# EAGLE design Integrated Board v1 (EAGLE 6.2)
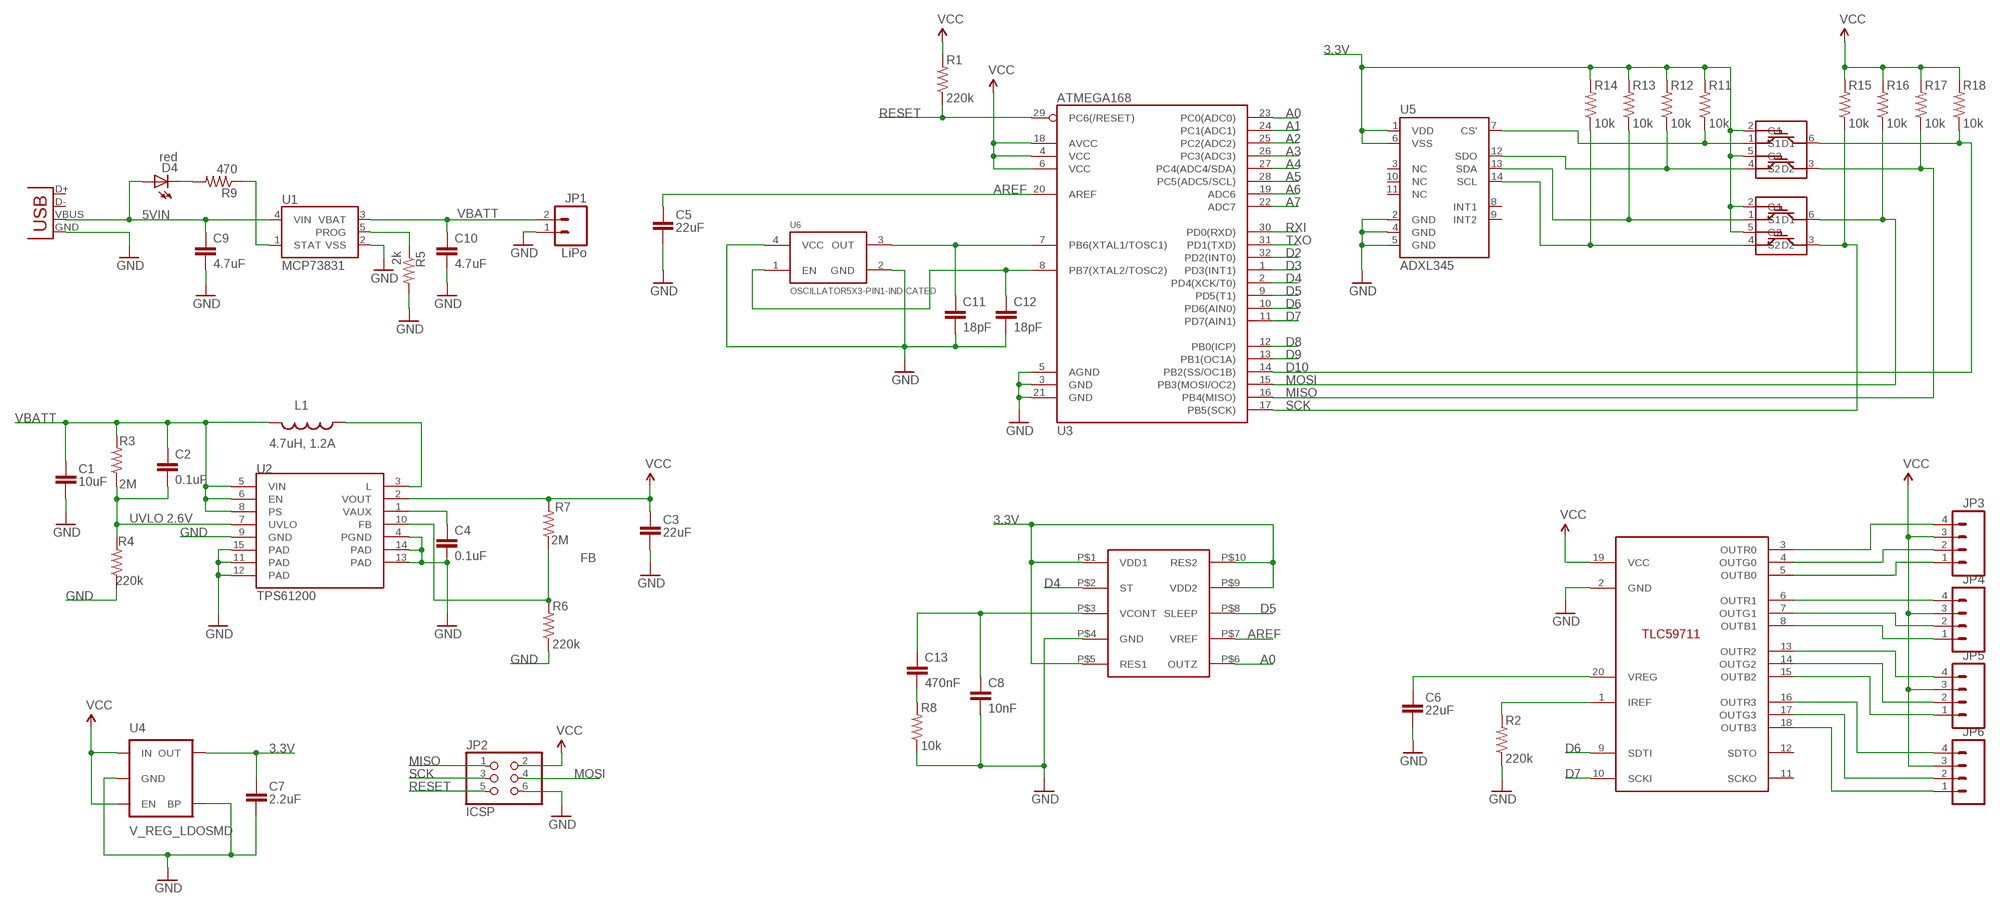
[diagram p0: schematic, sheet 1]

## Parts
C1  10uF  CAP0603  [0603]
C2  0.1uF  CAP0603-CAP  [0603-CAP]
C3  22uF  CAP0805  [0805]
C4  0.1uF  CAP0603-CAP  [0603-CAP]
C5  22uF  CAP0805  [0805]
C6  22uF  CAP0805  [0805]
C7  2.2uF  CAP0603  [0603]
C8  10nF  CAP0603-CAP  [0603-CAP]
C9  4.7uF  CAP0603-CAP  [0603-CAP]
C10  4.7uF  CAP0603-CAP  [0603-CAP]
C11  18pF  CAP0603-CAP  [0603-CAP]
C12  18pF  CAP0603-CAP  [0603-CAP]
C13  470nF  CAP0603-CAP  [0603-CAP]
D4  red  LED0603  [LED-0603]
JP1  LiPo  M02-JST-2MM-SMT  [JST-2-SMD]
JP2  ICSP  PINHD-2X3  [2X03]
JP3  M04PTH  [1X04]
JP4  M04PTH  [1X04]
JP5  M04PTH  [1X04]
JP6  M04PTH  [1X04]
L1  4.7uH, 1.2A  INDUCTOR.  [CDRH2D09]
R1  220k  RESISTOR0603-RES  [0603-RES]
R2  220k  RESISTOR0603-RES  [0603-RES]
R3  2M  RESISTOR0603-RES  [0603-RES]
R4  220k  RESISTOR0603-RES  [0603-RES]
R5  2k  RESISTOR0603-RES  [0603-RES]
R6  220k  RESISTOR0603-RES  [0603-RES]
R7  2M  RESISTOR0603-RES  [0603-RES]
R8  10k  RESISTOR0603-RES  [0603-RES]
R9  470  RESISTOR0603-RES  [0603-RES]
R11  10k  RESISTOR0603-RES  [0603-RES]
R12  10k  RESISTOR0603-RES  [0603-RES]
R13  10k  RESISTOR0603-RES  [0603-RES]
R14  10k  RESISTOR0603-RES  [0603-RES]
R15  10k  RESISTOR0603-RES  [0603-RES]
R16  10k  RESISTOR0603-RES  [0603-RES]
R17  10k  RESISTOR0603-RES  [0603-RES]
R18  10k  RESISTOR0603-RES  [0603-RES]
U1  MCP73831  [SOT23-5]
U2  TPS61200  [QFN-10_PAD]
U3  ATMEGA168  [TQFP32-08]
U4  V_REG_LDOSMD  [SOT23-5]
U5  ADXL345  [LGA14]
U6  OSCILLATOR5X3-PIN1-INDICATED  [CRYSTAL-OSC-SMD-5X3]
U$1  TLC59711  [TSSOP20]
U$2  2N7002DW  [SOT363]
U$3  2N7002DW  [SOT363]
U$4  LY3100ALH  [LGA10]
X1  USB-MICROB  [USB-MICROB]

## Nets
3.3V: C7.1 R11.2 R12.2 R13.2 R14.2 U4.5(OUT) U5.1(VDD) U5.6(VSS) U$2.2(G1) U$2.5(G2) U$3.2(G1) U$3.5(G2) U$4.P$1(VDD1) U$4.P$5(RES1) U$4.P$9(VDD2) U$4.P$10(RES2)
5VIN: C9.1 D4.A U1.4(VIN) X1.VBUS
A0: U3.23(PC0(ADC0)) U$4.P$6(OUTZ)
A1: U3.24(PC1(ADC1))
A2: U3.25(PC2(ADC2))
A3: U3.26(PC3(ADC3))
A4: U3.27(PC4(ADC4/SDA))
A5: U3.28(PC5(ADC5/SCL))
A6: U3.19(ADC6)
A7: U3.22(ADC7)
AREF: C5.1 U3.20(AREF) U$4.P$7(VREF)
D2: U3.32(PD2(INT0))
D3: U3.1(PD3(INT1))
D4: U3.2(PD4(XCK/T0)) U$4.P$2(ST)
D5: U3.9(PD5(T1)) U$4.P$8(SLEEP)
D6: U3.10(PD6(AIN0)) U$1.9(SDTI)
D7: U3.11(PD7(AIN1)) U$1.10(SCKI)
D8: U3.12(PB0(ICP))
D9: U3.13(PB1(OC1A))
D10: R18.1 U3.14(PB2(SS/OC1B)) U$2.6(D1)
FB: R6.2 R7.1 U2.10(FB)
GND: C1.2 C3.2 C4.2 C5.2 C6.2 C7.2 C8.2 C9.2 C10.2 C11.2 C12.2 JP1.1 JP2.6 R2.1 R4.1 R5.2 R6.1 R8.1 U1.2(VSS) U2.4(PGND) U2.9(GND) U2.11(PAD) U2.12(PAD) U2.13(PAD) U2.14(PAD) U2.15(PAD) U3.3(GND) U3.5(AGND) U3.21(GND) U4.2(GND) U4.4(BP) U5.2(GND) U5.4(GND) U5.5(GND) U6.2(GND) U6.4(VCC) U$1.2(GND) U$4.P$4(GND) X1.GND
MISO: JP2.1 R17.1 U3.16(PB4(MISO)) U$2.3(D2)
MOSI: JP2.4 R16.1 U3.15(PB3(MOSI/OC2)) U$3.6(D1)
N$1: C4.1 U2.1(VAUX)
N$2: L1.P$1 U2.3(L)
N$3: C11.1 U3.7(PB6(XTAL1/TOSC1)) U6.3(OUT)
N$5: C13.2 R8.2
N$6: C6.1 U$1.20(VREG)
N$7: R2.2 U$1.1(IREF)
N$8: D4.C R9.2
N$10: R11.1 U5.7(CS') U$2.1(S1)
N$11: R5.1 U1.5(PROG)
N$12: R12.1 U5.12(SDO) U$2.4(S2)
N$13: R13.1 U5.13(SDA) U$3.1(S1)
N$14: R9.1 U1.1(STAT)
N$15: R14.1 U5.14(SCL) U$3.4(S2)
N$16: JP4.4(B) U$1.6(OUTR1)
N$17: JP4.2(R) U$1.7(OUTG1)
N$18: JP4.1(COM) U$1.8(OUTB1)
N$19: JP5.4(B) U$1.13(OUTR2)
N$20: JP5.2(R) U$1.14(OUTG2)
N$21: JP5.1(COM) U$1.15(OUTB2)
N$22: JP6.4(B) U$1.16(OUTR3)
N$23: JP6.2(R) U$1.17(OUTG3)
N$24: JP6.1(COM) U$1.18(OUTB3)
N$25: JP3.1(COM) U$1.5(OUTB0)
N$26: JP3.2(R) U$1.4(OUTG0)
N$27: JP3.4(B) U$1.3(OUTR0)
N$28: C12.1 U3.8(PB7(XTAL2/TOSC2)) U6.1(EN)
N$30: C8.1 C13.1 U$4.P$3(VCONT)
RESET: JP2.5 R1.1 U3.29(PC6(/RESET))
RXI: U3.30(PD0(RXD))
SCK: JP2.3 R15.1 U3.17(PB5(SCK)) U$3.3(D2)
TXO: U3.31(PD1(TXD))
UVLO: C2.2 R3.1 R4.2 U2.7(UVLO)
VBATT: C1.1 C2.1 C10.1 JP1.2 L1.P$2 R3.2 U1.3(VBAT) U2.5(VIN) U2.6(EN) U2.8(PS)
VCC: C3.1 JP2.2 JP3.3(G) JP4.3(G) JP5.3(G) JP6.3(G) R1.2 R7.2 R15.2 R16.2 R17.2 R18.2 U2.2(VOUT) U3.4(VCC) U3.6(VCC) U3.18(AVCC) U4.1(IN) U4.3(EN) U$1.19(VCC)
Unconnected: U5.3(NC) U5.8(INT1) U5.9(INT2) U5.10(NC) U5.11(NC) U$1.11(SCKO) U$1.12(SDTO) X1.D+ X1.D-

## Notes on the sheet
- UVLO 2.6V

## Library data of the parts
C1 C3 C5-C7 = CH_passive:CAP: Capacitor
C2 C4 C8-C13 = SparkFun:CAP: Capacitor
D4 = SparkFun:LED: LEDs
JP1 = SparkFun:M02: Header 2
JP2 = SparkFun:PINHD-2X3: PIN HEADER
JP3-JP6 = SparkFun:M04: Header 4 Standard 4-pin 0.1" header. Use with straight break away headers (SKU : PRT-00116), right angle break away headers (PRT-00553), swiss pins (PRT-00743), machine pins (PRT-00117), and female headers (PRT-00115). Molex polarized connector foot print use with SKU : PRT-08231 with associated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
L1 = SparkFun:INDUCTOR: Inductors
R1-R9 R11-R18 = SparkFun:RESISTOR: Resistor
U1 = SparkFun:MCP73831: Microchip's MCP73831 Miniature single cell, fully integrated Li-Ion, Li-polymer charge management controller http://ww1.microchip.com/downloads/en/DeviceDoc/21984a.pdf
U2 = SparkFun:TPS61200: DC to DC Booster
U3 = SparkFun:ATMEGA168
U4 = SparkFun:V_REG_LDO: Voltage Regulator LDO Standard 150mA LDO voltage regulator in SOT-23 layout. Micrel part MIC5205. BP (by-pass) pin is used to lower output noise with 470pF cap.
U5 = SparkFun:ADXL345
U6 = SparkFun:OSCILLATOR
U$1 = SparkFun:TLC59711: TLC59711 RGB LED controller
U$2 U$3 = SparkFun:2N7002DW
U$4 = SparkFun:LY3100ALH
X1 = SparkFun:USB: USB Connectors USB-B-PTH is fully proven SKU : PRT-00139 USB-miniB is fully proven SKU : PRT-00587 USB-A-PCB is untested. USB-A-H is throughly reviewed, but untested. Spark Fun Electronics SKU : PRT-00437 USB-B-SMT is throughly reviewed, but untested. Needs silkscreen touching up. USB-A-S has not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

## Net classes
0 default: width 0.203 mm
1 vcc: width 0.254 mm

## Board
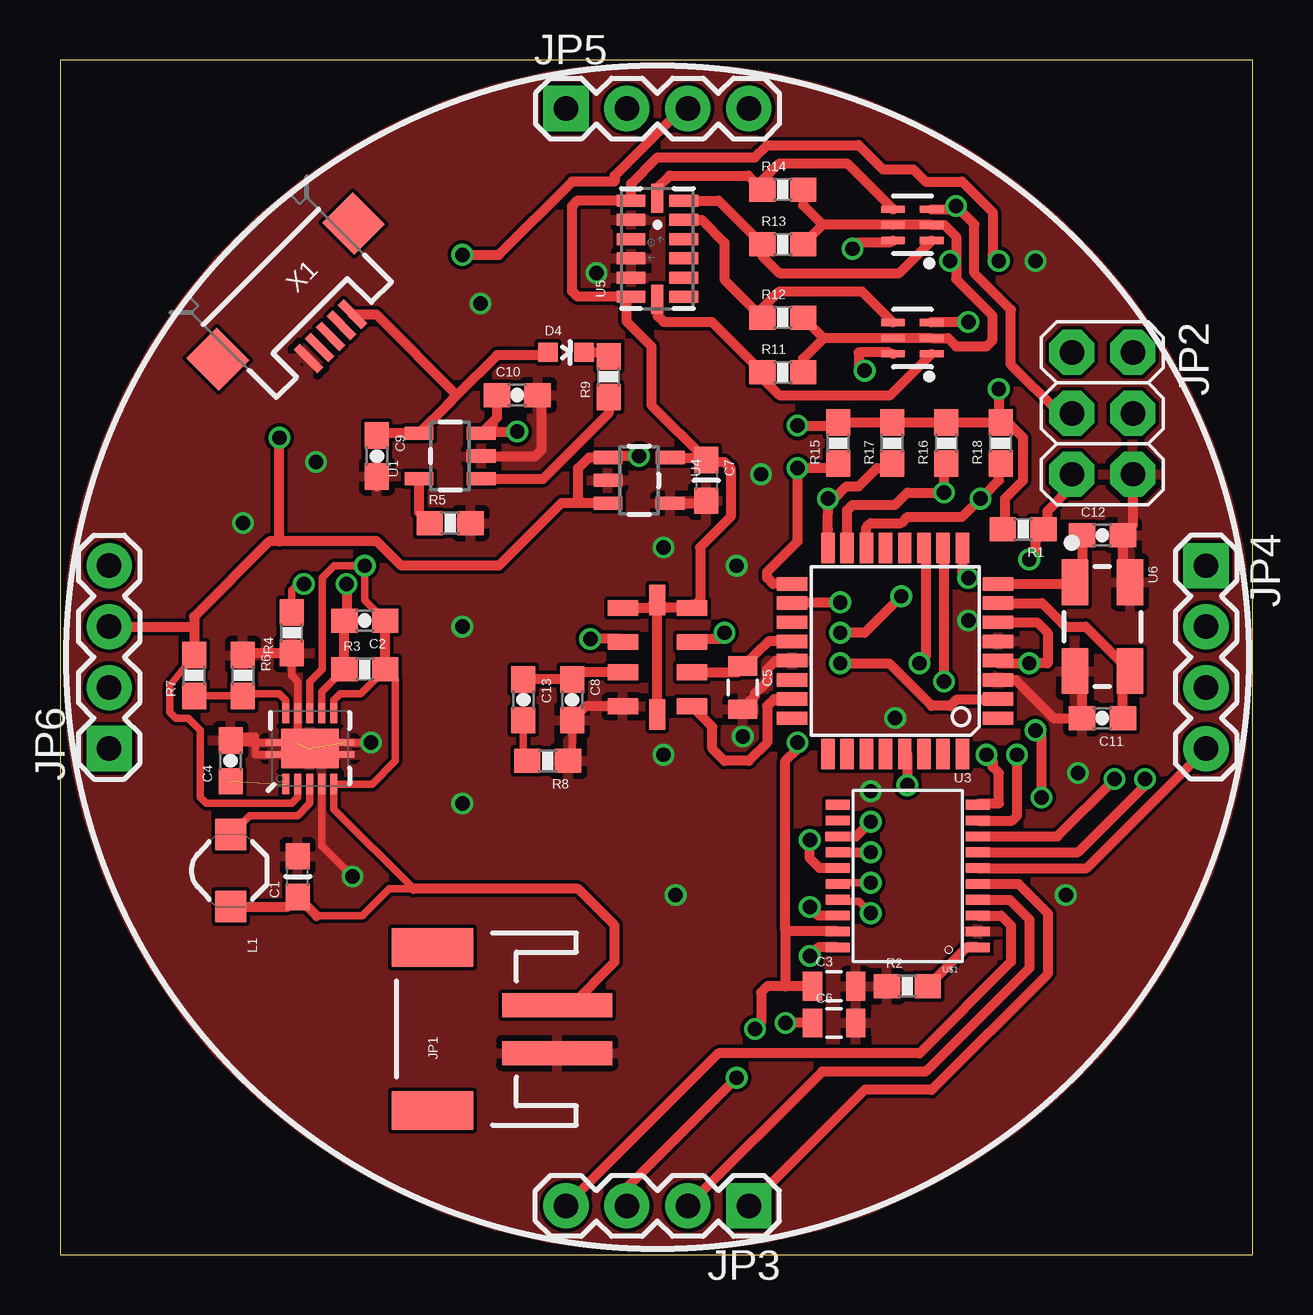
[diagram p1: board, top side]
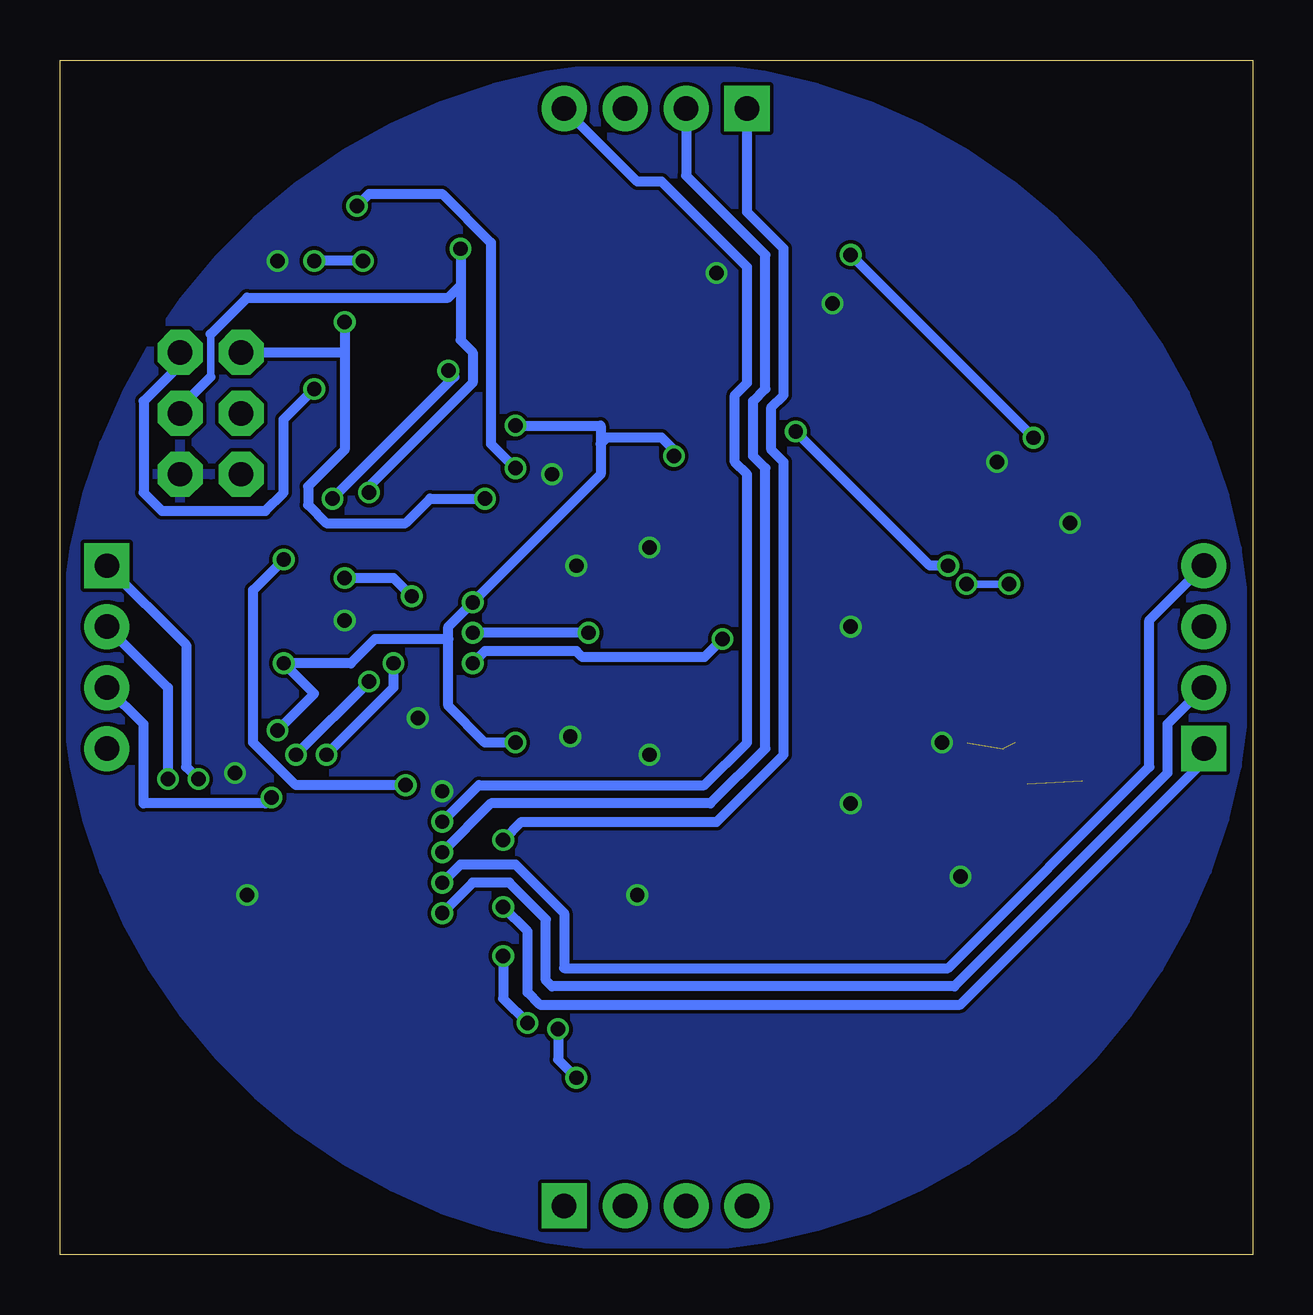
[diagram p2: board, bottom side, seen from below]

Size 49.71 x 49.77 mm. Coordinates in mm from the lower left corner, seen from the top.
Outline: 0,0 49.71,0 49.71,49.77 0,49.77 0,0
Copper layers (1*16): Top 0.035mm / dielectric 1.5mm / Bottom 0.035mm
Design rules: minimum track width 6mil, minimum drill 12mil, track to track 6mil, track to pad 6mil, pad to pad 6mil, via to via 6mil, smd to smd 0mil, copper to edge 10mil, drill to drill 10mil, minimum pad ring 10mil, minimum via ring 6mil, stop-mask expansion 2mil, vias tented up to drill 100mil, thermal gap 10mil

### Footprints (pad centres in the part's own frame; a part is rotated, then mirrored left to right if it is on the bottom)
0603 = smd 1.1 x 1: 1 -0.85,0; 2 0.85,0
0603-CAP = smd 1.1 x 1: 1 -0.85,0; 2 0.85,0
0805 = smd 0.8 x 1.2: 1 -0.9,0; 2 0.9,0
LED-0603 = smd 0.8 x 0.8: A 0,-0.75; C 0,0.75
JST-2-SMD = smd 1 x 4.6: 1 -1,-3.7; 2 1,-3.7 | smd 1.6 x 3.4: NC1 -3.4,1.5; NC2 3.4,1.5
2X03 = drill 1.016 pad 1.88 octagon: 1 -2.54,-1.27; 2 -2.54,1.27; 3 0,-1.27; 4 0,1.27; 5 2.54,-1.27; 6 2.54,1.27
1X04 = drill 1.016 pad 1.88 square: 1 0,0 | drill 1.016 pad 1.88: 2 2.54,0; 3 5.08,0; 4 7.62,0
CDRH2D09 = smd 1.3 x 1.3: P$1 -1.5,0; P$2 1.5,0
0603-RES = smd 1.1 x 1: 1 -0.85,0; 2 0.85,0
SOT23-5 = smd 0.55 x 1.2: 1 -0.95,-1.3; 2 0,-1.3; 3 0.95,-1.3; 4 0.95,1.3; 5 -0.95,1.3
QFN-10_PAD = smd 0.297 x 0.85: 1 -1,-1.475; 2 -0.5,-1.475; 3 0,-1.475; 4 0.5,-1.475; 5 1,-1.475; 6 1,1.475; 7 0.5,1.475; 8 0,1.475; 9 -0.5,1.475; 10 -1,1.475 | smd 0.7 x 0.28: 11 -1.5,0.25; 12 -1.5,-0.25; 13 1.5,0.25; 14 1.5,-0.25 | smd 2.4 x 1.65: 15 0,0
TQFP32-08 = smd 1.27 x 0.559: 1 -4.293,2.8; 2 -4.293,2; 3 -4.293,1.2; 4 -4.293,0.4; 5 -4.293,-0.4; 6 -4.293,-1.2; 7 -4.293,-2; 8 -4.293,-2.8; 17 4.293,-2.8; 18 4.293,-2; 19 4.293,-1.2; 20 4.293,-0.4; 21 4.293,0.4; 22 4.293,1.2; 23 4.293,2; 24 4.293,2.8 | smd 0.559 x 1.27: 9 -2.8,-4.293; 10 -2,-4.293; 11 -1.2,-4.293; 12 -0.4,-4.293; 13 0.4,-4.293; 14 1.2,-4.293; 15 2,-4.293; 16 2.8,-4.293; 25 2.8,4.293; 26 2,4.293; 27 1.2,4.293; 28 0.4,4.293; 29 -0.4,4.293; 30 -1.2,4.293; 31 -2,4.293; 32 -2.8,4.293
LGA14 = smd 0.5 x 1.2: 1 2,1.1; 2 1.2,1.1; 3 0.4,1.1; 4 -0.4,1.1; 5 -1.2,1.1; 6 -2,1.1; 8 -2,-1.1; 9 -1.2,-1.1; 10 -0.4,-1.1; 11 0.4,-1.1; 12 1.2,-1.1; 13 2,-1.1 | smd 1.2 x 0.5: 7 -2.1,0; 14 2.1,0
CRYSTAL-OSC-SMD-5X3 = smd 1.9 x 1.1: 1 -1.85,-1.15; 2 1.85,-1.15; 3 1.85,1.15; 4 -1.85,1.15
TSSOP20 = smd 1 x 0.4: 1 -2.937,2.693; 2 -2.937,2.032; 3 -2.937,1.372; 4 -2.937,0.712; 5 -2.937,0.051; 6 -2.937,-0.609; 7 -2.937,-1.27; 8 -2.943,-1.93; 9 -2.937,-2.59; 10 -2.937,-3.251; 11 2.905,-3.251; 12 2.905,-2.59; 13 2.911,-1.93; 14 2.905,-1.27; 15 2.905,-0.609; 16 2.905,0.051; 17 2.905,0.712; 18 2.905,1.372; 19 2.905,2.032; 20 2.905,2.693
SOT363 = smd 0.3 x 0.99: 1 -0.65,-0.8; 2 0,-0.8; 3 0.65,-0.8; 4 0.65,0.81; 5 0,0.81; 6 -0.65,0.81
LGA10 = smd 1.27 x 0.66: P$1 -1.435,2.05; P$2 -1.435,0.635; P$3 -1.435,-0.635; P$4 -1.435,-2.05; P$6 1.435,-2.05; P$7 1.435,-0.635; P$8 1.435,0.635; P$9 1.435,2.05 | smd 0.66 x 1.27: P$5 0,-2.385; P$10 0,2.385
USB-MICROB = smd 0.35 x 1.4: D+ 0,2.65; D- -0.65,2.65; GND 1.3,2.65; ID 0.65,2.65; VBUS -1.3,2.65 | smd 1.8 x 1.9: MT1 -4,0; MT2 4,0

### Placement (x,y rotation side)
C1  9.91,15.75 90 top
C2  12.7,26.42 180 top
C3  32.26,11.18 0 top
C4  7.11,20.57 90 top
C5  28.45,23.62 270 top
C6  32.26,9.65 0 top
C7  26.92,32.26 270 top
C8  21.34,23.11 270 top
C9  13.21,33.27 270 top
C10  19.05,35.81 0 top
C11  43.43,22.35 180 top
C12  43.43,29.97 0 top
C13  19.3,23.11 270 top
D4  21.08,37.59 270 top
JP1  17.02,9.4 90 top
JP2  43.43,35.05 270 top
JP3  28.7,2.03 180 top
JP4  47.75,28.7 270 top
JP5  21.08,47.75 0 top
JP6  2.04,21.09 90 top
L1  7.11,16 270 top
R1  40.13,30.23 180 top
R2  35.31,11.18 0 top
R3  12.7,24.38 0 top
R4  9.65,25.91 90 top
R5  16.26,30.48 0 top
R6  7.62,24.13 270 top
R7  5.59,24.13 90 top
R8  20.32,20.57 180 top
R9  22.86,36.58 90 top
R11  30.12,36.75 0 top
R12  30.12,39.04 0 top
R13  30.12,42.09 0 top
R14  30.12,44.37 0 top
R15  32.43,33.81 90 top
R16  36.93,33.81 90 top
R17  34.68,33.81 90 top
R18  39.19,33.81 90 top
U1  16.26,33.27 90 top
U2  10.41,21.08 0 top
U3  34.8,25.15 180 top
U4  24.13,32.26 270 top
U5  24.89,41.91 90 top
U6  43.43,26.16 270 top
U$1  35.31,15.49 180 top
U$2  35.52,38.18 90 top
U$3  35.52,42.9 90 top
U$4  24.89,24.89 0 top
X1  9.4,40.13 225 top

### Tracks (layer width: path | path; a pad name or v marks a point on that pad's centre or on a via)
3.3V  (via drill 0.6)
  Top 0.406: 31.78,42.9 U$3.5 U$3.2 36.85,42.9 37.34,42.42 37.34,41.4 | 31.78,42.9 R13.2 | R14.2 30.97,43.72 31.78,42.9 | 31.82,38.18 U$2.5 U$2.2 37,38.18 37.34,37.85 38.61,37.85 38.86,38.1 38.86,39.12 37.34,40.64 37.34,41.4 | 31.82,38.18 R12.2 | R11.2 30.97,37.33 31.82,38.18 | U$4.P$9 25.23,26.94 U$4.P$10 | U$4.P$1 24.56,26.94 U$4.P$10 | U$4.P$5 U$4.P$10 | U4.5 26.82,33.21 C7.1 | U$4.P$9 26.33,27.09 | C7.1 27.01,33.02 27.69,33.02 27.94,32.77 27.94,30.73 26.67,29.46 26.67,27.29 U$4.P$9 | v39.12,41.4 38.86,41.66 38.86,43.43 37.59,44.7 36.07,44.7 35.56,45.21 34.29,45.21 33.27,46.23 29.46,46.23 28.96,45.72 24.89,45.72 23.79,44.62 U5.1 21.56,43.91 21.34,43.69 21.34,40.13 21.56,39.91 U5.6 23.62,39.74 23.62,38.86 24.64,37.85 24.64,35.39 C7.1 | 37.34,41.4 v37.08,41.4
  Bottom 0.406: v37.08,41.4 v39.12,41.4
5VIN
  Top 0.406: 16.54,35.81 16.15,35.41 U1.4 13.31,34.22 C9.1 | D4.A 20.22,37.48 18.21,37.48 16.54,35.81 | X1.VBUS 13.17,39.18 16.54,35.81
A0
  Top 0.406: U3.23 29.75,23.15 29.46,22.86 29.46,21.34 28.7,20.57 27.69,20.57 27.18,21.08 27.18,21.99 U$4.P$6
AREF
  Top 0.406: U$4.P$7 28.23,24.26 C5.1 29.52,25.55 U3.20
D4  (via drill 0.6)
  Top 0.406: U3.2 38.86,23.11 37.34,23.11 37.08,22.86 36.32,22.86 34.54,24.64 v32.51,24.64 | v22.1,25.65 23.37,25.65 U$4.P$2
  Bottom 0.406: v32.51,24.64 32,25.15 28.19,25.15 27.94,24.89 22.86,24.89 v22.1,25.65
D5  (via drill 0.6)
  Top 0.406: v32.51,25.91 33.53,25.91 v35.05,27.43 | v37.85,28.19 37.59,28.45 37.59,29.21 U3.9 | v27.69,25.91 27.43,25.65 26.42,25.65 U$4.P$8
  Bottom 0.406: v35.05,27.43 35.81,28.19 v37.85,28.19 | v27.69,25.91 v32.51,25.91
D6  (via drill 0.6)
  Top 0.406: U3.10 36.83,29.21 v36.83,23.88 | U$1.9 39.67,18.08 39.88,18.29 v39.88,20.83
  Bottom 0.406: v36.83,23.88 v39.88,20.83
D7  (via drill 0.6)
  Top 0.406: U$1.10 38.35,18.8 39.12,18.8 39.12,20.07 38.86,20.32 38.86,20.57 v38.61,20.83 | U3.11 36.07,29.21 36.07,24.89 v35.81,24.64
  Bottom 0.406: v38.61,20.83 35.81,23.62 v35.81,24.64
D10  (via drill 0.6)
  Top 0.406: U$2.6 34.54,37.59 33.27,37.59 33.27,36.83 v33.53,36.83 | 39.38,32.77 R18.1 39.12,32.89 39.12,32.26 38.48,31.62 | 38.48,31.62 37.59,30.73 35.31,30.73 35.05,30.48 33.78,30.48 33.6,30.3 U3.14 | v38.35,31.5 38.35,31.75 38.48,31.62
  Bottom 0.406: v38.35,31.5 33.27,36.58 v33.53,36.83
FB
  Top 0.305: R7.1 R6.2 7.71,23.37 9.14,23.37 9.41,23.1 U2.10
GND  (via drill 0.6)  (2 unrouted)
  Top 0.305: C8.2 21.34,20.74 R8.1 | 13.21,32 12.95,32 | 9.91,24.8 R4.1 | 9.57,24.98 R4.1 | U2.11 8.13,21.33 8.13,21.34 | 8.13,21.34 7.11,21.34 C4.2 7.11,21.59 8.13,21.59 8.13,20.83 U2.12 | 8.13,21.34 9.91,21.34 U2.9 9.91,23.87 9.65,24.13 R4.1 | U2.13 v12.95,21.33 v12.95,21.34 | U2.4 10.91,17.03 v12.19,15.75
  Top 0.406: U$4.P$4 21.91,22.84 C8.2 | U6.4 44.28,28.31 C12.2 44.7,30.39 JP2.6 | U6.2 42.58,24.01 C11.2 41.4,22.35 39.81,23.95 U3.3 | C7.2 26.82,31.31 U4.4 25.91,31.24 | U1.2 19.81,33.27 20.07,33.53 20.07,35.65 C10.2 | R5.2 16.76,30.48 | 29.83,24.75 29.46,24.38 29.46,23.88 28.96,23.37 28.96,23.28 C5.2 | 13.21,32.51 C9.2 13.21,32 | R4.1 7.7,25.06 R6.1
  other vias: 33.78,19.3 28.45,21.59 25.15,20.83 25.65,14.99 16.76,18.8 16.76,26.16 25.15,29.46 17.53,39.62 22.35,40.89 37.85,26.42 34.8,22.35 10.67,33.02 42.42,20.07 28.19,28.7 40.64,41.4 41.91,14.99 7.62,30.48 29.21,32.51
  pour Top: 0.25,24.89 arc-90 24.89,49.53 arc-90 49.53,24.89 arc-90 24.89,0.25 arc-90
  pour Bottom: 0.25,24.89 arc-90 24.89,49.53 arc-90 49.53,24.89 arc-90 24.89,0.25 arc-90
MISO  (via drill 0.6)
  Top 0.406: 34.8,32.77 R17.1 34.48,32.77 34.04,32.77 33.27,32 32.77,32 32.26,31.5 v32,31.5 32,30.22 U3.16 | v37.85,38.86 36.32,38.86 U$2.3
  Bottom 0.406: v32,31.5 34.29,31.5 35.31,30.48 38.61,30.48 39.37,31.24 39.37,32 37.85,33.53 37.85,37.59 | v37.85,38.86 37.85,37.59 | JP2.1 37.85,37.59
MOSI  (via drill 0.6)
  Top 0.406: U$3.6 34.54,42.16 33.27,42.16 v33.02,41.91 33.02,41.66 | R16.1 36.83,32.77 v36.83,31.75 35.31,31.75 34.8,31.24 33.02,31.24 32.8,31.02 U3.15
  Bottom 0.305: JP2.4 44.7,35.31 | 43.43,36.58 43.43,38.35
  Bottom 0.406: v33.02,41.91 33.02,40.39 | 33.02,40.39 33.02,38.1 32.51,37.59 32.51,36.32 36.83,32 v36.83,31.75 | 44.7,35.31 43.43,36.58 | 43.43,38.35 41.91,39.88 33.53,39.88 33.02,40.39
N$1  (1 unrouted)
N$2
  Top 0.305: U2.3 10.41,18.8 9.91,18.29 7.9,18.29 L1.P$1
N$3
  Top 0.406: U3.7 40.93,27.15 41.91,26.16 42.73,26.16 U6.3 44.28,24.01 C11.1
N$5
  Top 0.305: C13.2 19.3,20.74 R8.2
N$6  (via drill 0.6)
  Top 0.406: U$1.20 31.6,12.8 v31.24,12.45 | C6.1 v30.23,9.65
  Bottom 0.406: v31.24,12.45 31.24,10.67 v30.23,9.65
N$7
  Top 0.406: U$1.1 37.78,12.8 R2.2
N$8
  Top 0.406: D4.C 22.95,37.59 R9.2
N$10
  Top 0.406: U$2.1 34.6,35.81 29.97,35.81 29.27,36.52 R11.1 27.16,38.86 25.15,38.86 24.89,39.12 U5.7
N$11
  Top 0.406: U1.5 14.96,30.93 R5.1
N$12
  Top 0.406: U$2.4 33.41,40.13 29.97,40.13 29.27,39.43 R12.1 27.69,40.62 27.69,42.16 26.74,43.11 U5.12
N$13
  Top 0.406: U5.13 27.45,43.91 R13.1 29.27,41.6 29.97,40.89 34.96,40.89 U$3.1
N$14
  Top 0.406: U1.1 20.13,32.32 22.86,35.05 R9.1
N$15
  Top 0.406: U5.14 24.89,44.45 25.4,44.96 28.68,44.96 R14.1 29.27,44.76 29.97,45.47 32.8,45.47 U$3.4
N$16
  Top 0.406: U$1.6 42.77,16.1 JP4.4
N$17  (via drill 0.6)
  Top 0.406: U$1.7 38.35,16.76 42.42,16.76 45.21,19.56 v45.21,19.81
  Bottom 0.406: JP4.2 45.21,23.62 v45.21,19.81
N$18  (via drill 0.6)
  Top 0.406: U$1.8 41.55,17.42 v43.94,19.81
  Bottom 0.406: JP4.1 44.45,25.4 44.45,20.32 v43.94,19.81
N$19  (via drill 0.6)
  Top 0.406: v33.78,18.03 33.17,17.42 U$1.13
  Bottom 0.406: v33.78,18.03 32.26,19.56 22.86,19.56 21.08,21.34 21.08,32.51 21.59,33.02 21.59,35.81 21.08,36.32 21.08,41.15 24.64,44.7 25.65,44.7 JP5.4
N$20  (via drill 0.6)
  Top 0.406: v33.78,16.76 32.51,16.76 U$1.14
  Bottom 0.406: JP5.2 23.62,44.96 20.32,41.66 20.32,36.07 20.83,35.56 20.83,33.27 20.32,32.77 20.32,21.08 22.61,18.8 31.75,18.8 v33.78,16.76
N$21  (via drill 0.6)
  Top 0.406: U$1.15 31.65,16.1 31.24,16.51 v31.24,17.27
  Bottom 0.406: v31.24,17.27 30.48,18.03 22.35,18.03 19.56,20.83 19.56,33.02 20.07,33.53 20.07,35.31 19.56,35.81 19.56,41.91 21.08,43.43 JP5.1
N$22  (via drill 0.6)
  Top 0.305: U$1.16 32.51,15.49 v33.78,15.49
  Bottom 0.406: v33.78,15.49 33.02,16.26 30.73,16.26 28.7,14.22 28.7,11.94 12.7,11.94 4.32,20.32 4.32,26.43 JP6.4
N$23  (via drill 0.6)
  Top 0.305: U$1.17 32.51,14.73 33.27,14.73 v33.78,14.22
  Bottom 0.406: v33.78,14.22 32.51,15.49 30.99,15.49 29.46,13.97 29.46,11.43 29.21,11.18 12.45,11.18 3.56,20.07 3.56,22.11 JP6.2
N$24  (via drill 0.6)
  Top 0.406: U$1.18 31.6,14.12 v31.24,14.48
  Bottom 0.305: v31.24,14.48 31.24,14.22
  Bottom 0.406: v31.24,14.48 30.23,13.46 30.23,10.92 29.72,10.41 12.19,10.41 2.04,20.56 JP6.1
N$25
  Top 0.406: JP3.1 33.53,6.86 36.32,6.86 41.15,11.68 41.15,14.22 39.93,15.44 U$1.5
N$26
  Top 0.406: JP3.2 31.75,7.62 36.07,7.62 40.39,11.94 40.39,13.97 39.57,14.78 U$1.4
N$27
  Top 0.406: JP3.4 27.43,8.38 35.81,8.38 39.62,12.19 39.62,13.72 39.22,14.12 U$1.3
N$28
  Top 0.406: U3.8 42.22,27.95 U6.1 42.58,28.31 C12.1
N$30
  Top 0.406: C13.1 C8.1 21.63,24.26 U$4.P$3
RESET  (via drill 0.6)
  Top 0.406: JP2.5 42.16,32 41.15,30.99 41.15,30.23 R1.1 40.89,30.23 40.89,29.97 40.64,29.72 40.64,28.96 40.39,28.7 v40.39,28.96 | v35.31,19.56 35.31,20.83 U3.29
  Bottom 0.406: v40.39,28.96 41.66,27.69 41.66,21.34 39.88,19.56 v35.31,19.56
SCK  (via drill 0.6)
  Top 0.406: R15.1 32.26,32.77 v30.73,32.77 30.73,29.72 29.46,28.45 29.46,28.19 29.72,27.94 29.72,27.95 U3.17 | U$3.3 37.22,43.55 v37.34,43.69 38.1,42.93 38.1,40.89 39.62,39.37 39.62,37.08 41.66,35.05 JP2.3
  Bottom 0.406: v30.73,32.77 31.75,33.78 31.75,42.16 33.78,44.2 36.83,44.2 v37.34,43.69
UVLO  (via drill 0.6)
  Top 0.305: R3.1 10.91,23.45 U2.7 | v10.16,27.94 9.91,27.94 9.65,27.69 R4.2
  Top 0.406: R3.1 C2.2 11.94,26.5 v11.94,27.94
  Bottom 0.305: v10.16,27.94 v11.94,27.94
VBATT  (via drill 0.6)
  Top 0.305: U2.6 11.41,23.1 11.68,23.37 12.53,23.37 R3.2 13.97,23.96 13.97,20.57 13,19.61 U2.5 11.41,18.56 14.73,15.24 13.72,15.24 12.59,14.11 10.69,14.11 | C2.1 12.7,27.27 v12.7,28.7 11.43,28.7 10.92,28.19 10.92,24.38 10.41,23.88 U2.8
  Top 0.406: R3.2 C2.1 | C10.1 18.2,34.87 17.95,34.62 | 17.95,34.62 U1.3 | 10.69,14.11 C1.1 9.51,14.5 L1.P$2 | 17.95,34.62 18.03,34.54 18.03,34.29 v19.05,34.29 | JP1.2 21.32,10.4 23.11,12.19 23.11,13.72 21.59,15.24 14.73,15.24
  Bottom 0.406: v19.05,34.29 13.46,28.7 v12.7,28.7
VCC  (via drill 0.6)
  Top 0.305: U2.2 9.91,19.06 9.65,18.8 6.1,18.8 5.84,19.05 5.84,21.84 5.33,22.35 4.83,22.35 4.57,22.61 4.57,23.71 R7.2
  Top 0.406: R18.2 R16.2 R17.2 R15.2 | 21.78,31.31 U4.3 22.86,31.24 | 21.78,31.31 21.59,31.5 21.59,32.77 22.03,33.21 U4.1 22.9,33.27 v24.13,33.27 | 21.78,31.31 20.89,31.31 18.29,28.7 14.22,28.7 13.21,29.72 9.14,29.72 | 32.51,34.8 R15.2 | v30.73,34.54 32.31,34.54 R15.2 | U3.4 39.12,24.64 v40.39,24.64 41.15,24.64 41.15,25.91 40.71,26.35 U3.6 | U3.18 30.73,27.18 32.26,27.18 32.51,27.43 v32.51,27.18 | 30.23,13.46 30.23,11.18 | C3.1 30.23,11.18 | 30.23,13.46 32.26,13.46 U$1.19 30.23,13.46 | 5.59,26.16 5.59,26.58 8.72,29.72 9.14,29.72 | 5.59,26.16 R7.2 | JP6.3 5.58,26.16 5.59,26.16 | R18.2 39.37,34.8 40.13,34.04 40.13,32.26 39.37,31.5 39.37,30.23 R1.2 | JP5.3 25.91,47.75 23.11,44.96 23.11,44.7 21.34,44.7 18.29,41.66 v16.76,41.66 | v39.12,36.07 39.12,34.73 R18.2 | 30.23,13.46 | 30.23,13.46 30.23,20.57 30.73,21.08 v30.73,21.34 | v28.96,9.4 29.21,9.65 29.21,10.92 29.46,11.18 30.23,11.18 | JP3.3 23.62,2.79 v28.19,7.37 | v40.89,19.05 40.89,21.59 v40.64,21.84 | 9.14,29.72 v9.14,34.04
  Bottom 0.406: v30.73,34.54 27.18,34.54 27.18,33.78 | 27.18,33.78 27.18,32.51 v32.51,27.18 33.53,26.16 33.53,25.65 | v24.13,33.27 24.13,33.53 24.64,34.04 26.92,34.04 27.18,33.78 | JP2.2 44.7,37.08 46.23,35.56 46.23,31.75 45.47,30.99 41.15,30.99 40.39,31.75 40.39,34.8 v39.12,36.07 | v30.73,21.34 32,21.34 33.53,22.86 33.53,25.65 | v28.19,7.37 28.96,8.13 v28.96,9.4 | v40.64,21.84 39.12,23.37 v40.39,24.64 37.59,24.64 36.58,25.65 33.53,25.65 | JP4.3 46.23,22.1 46.23,18.8 41.15,18.8 v40.89,19.05 | v16.76,41.66 v9.14,34.04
